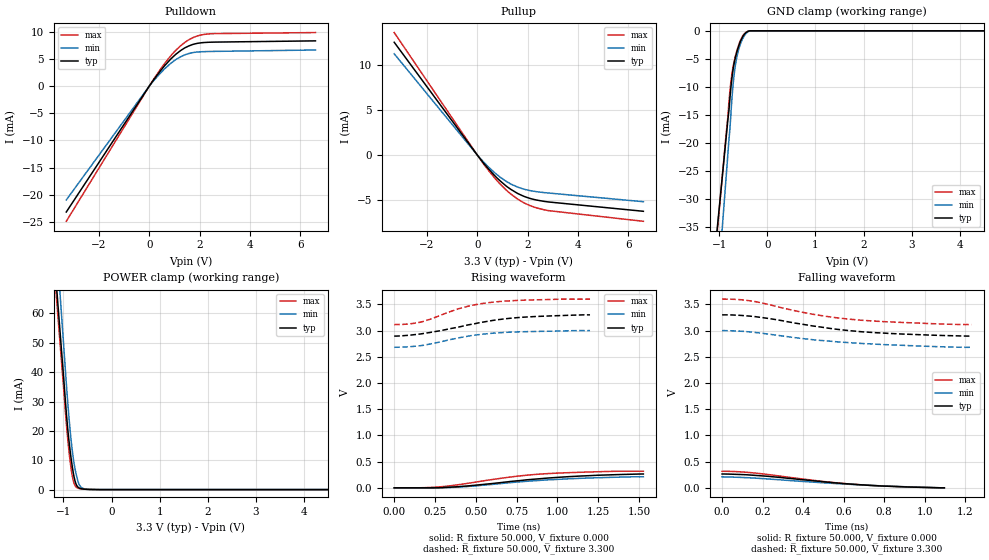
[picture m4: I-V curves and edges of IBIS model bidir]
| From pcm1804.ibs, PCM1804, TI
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[Model]   bidir
Model_type I/O
Vinl=8.000E-01
Vinh=2.000E+00
Vref=0.000E+00
Rref=1.000E+06
Cref=0.000E+00
Vmeas=1.650E+00
C_comp   8.900E-13   8.880E-13   8.930E-13
[Voltage Range]   3.300E+00   3.000E+00   3.600E+00
[POWER Clamp Reference]   3.300E+00   3.000E+00   3.600E+00
[GND Clamp Reference]   0.000E+00   0.000E+00   0.000E+00
[Pullup Reference]   3.300E+00   3.000E+00   3.600E+00
[Pulldown Reference]   0.000E+00   0.000E+00   0.000E+00
[Temperature Range]   25   70   -10
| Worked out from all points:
|   slope of the pulldown table from 0 to 0.495 V, typ, clamps not added: 160 ohm
|   slope of the pullup table from 0 to 0.495 V, typ, clamps not added: 292 ohm
|   GND clamp passes 1 mA (typ) near -0.51 V on its own axis
|   POWER clamp passes 1 mA (typ) near -0.71 V on its own axis
|   rising waveform, R_fixture 50.000, V_fixture 0.000: 20-80 % time 555ps typ, 530ps min, 454ps max; typ from 0 V to 0.264 V
|   falling waveform, R_fixture 50.000, V_fixture 0.000: 20-80 % time 459ps typ, 533ps min, 438ps max; typ from 0.264 V to 0 V
|   rising waveform, R_fixture 50.000, V_fixture 3.300: 20-80 % time 424ps typ, 337ps min, 298ps max; typ from 2.9 V to 3.3 V
|   falling waveform, R_fixture 50.000, V_fixture 3.300: 20-80 % time 445ps typ, 518ps min, 422ps max; typ from 3.3 V to 2.9 V
[GND Clamp]
-3.3V     -232.4mA   -302.2mA   -248.8mA
-860mV    -19.24mA   -26.33mA   -18.65mA
-820mV    -15.75mA   -21.82mA   -15.17mA
-800mV    -14.27mA   -19.5mA    -12.77mA
-780mV    -12.13mA   -17.61mA   -10.83mA
-760mV    -10.22mA   -15.02mA   -9.19mA
-720mV    -7.29mA    -10.23mA   -6.747mA
-660mV    -4.573mA   -5.874mA   -4.354mA
-560mV    -1.885mA   -2.334mA   -1.71mA
-480mV    -627.3uA   -874.5uA   -516.4uA
-400mV    -90.86uA   -152.2uA   -66.2uA
6.6V      0A         0A         0A
[Power Clamp]
-3.3V     522.9mA    587.4mA    513.2mA
-1.02V    43.15mA    54.89mA    39.38mA
-920mV    22.35mA    31.7mA     18.83mA
-880mV    15.84mA    23.62mA    12.3mA
-840mV    10.56mA    16.72mA    7.061mA
-800mV    6.176mA    11.23mA    3.341mA
-780mV    4.413mA    9.024mA    2.174mA
-740mV    1.98mA     5.539mA    938.8uA
-700mV    870.8uA    2.963mA    491.7uA
-620mV    272.2uA    601.8uA    212.3uA
-460mV    51.82uA    58.54uA    63.45uA
6.6V      0A         0A         0A
[Pullup]
-3.3V     12.56mA    11.28mA    13.64mA
20mV      -69.87uA   -65.87uA   -82.31uA
340mV     -1.204mA   -1.04mA    -1.32mA
700mV     -2.319mA   -1.99mA    -2.59mA
1.14V     -3.435mA   -2.915mA   -3.882mA
1.34V     -3.84mA    -3.241mA   -4.363mA
1.6V      -4.277mA   -3.569mA   -4.903mA
1.92V     -4.674mA   -3.856mA   -5.418mA
2.36V     -5.02mA    -4.089mA   -5.896mA
2.64V     -5.159mA   -4.183mA   -6.093mA
6.6V      -6.271mA   -5.204mA   -7.386mA
[Pulldown]
-3.3V     -23.19mA   -20.97mA   -24.9mA
120mV     803uA      694uA      882.4uA
480mV     3.018mA    2.567mA    3.335mA
800mV     4.717mA    3.968mA    5.266mA
1.06V     5.871mA    4.885mA    6.619mA
1.4V      6.994mA    5.719mA    7.996mA
1.7V      7.607mA    6.125mA    8.835mA
1.9V      7.85mA     6.255mA    9.209mA
2.36V     8.054mA    6.355mA    9.591mA
6.6V      8.311mA    6.63mA     9.839mA
[Rising Waveform]
R_fixture = 50.000
V_fixture = 0.000
V_fixture_min = 0.000
V_fixture_max = 0.000
|  time   V(typ)   V(min)   V(max)
0s        0V         0V         0V
177.5ps   0V         2.38uV     2.939mV
295ps     5.044mV    3.189mV    23.67mV
452.5ps   37.24mV    26.28mV    86.98mV
702.5ps   118.2mV    96.24mV    203mV
907.5ps   178.2mV    145.8mV    265.6mV
1.07ns    213.7mV    172.6mV    289.6mV
1.245ns   240mV      192.6mV    307.2mV
1.367ns   252.5mV    203.4mV    316.7mV
1.527ns   264.4mV    211.2mV    317.1mV
[Falling Waveform]
R_fixture = 50.000
V_fixture = 0.000
V_fixture_min = 0.000
V_fixture_max = 0.000
|  time   V(typ)   V(min)   V(max)
0s        264.4mV    211.2mV    317.1mV
82.5ps    255.9mV    200.7mV    307.1mV
152.5ps   241mV      188.1mV    286.3mV
232.5ps   218.1mV    167.9mV    251.3mV
457.5ps   132.4mV    107.1mV    140.6mV
550ps     97.82mV    84.85mV    101.4mV
647.5ps   68.31mV    64.06mV    68.22mV
760ps     41.25mV    42.63mV    41.76mV
852.5ps   25.49mV    28.29mV    27.12mV
1.097ns   0V         0V         0V
[Rising Waveform]
R_fixture = 50.000
V_fixture = 3.300
V_fixture_min = 3.000
V_fixture_max = 3.600
|  time   V(typ)   V(min)   V(max)
0s        2.895V     2.681V     3.115V
82.5ps    2.909V     2.69V      3.124V
162.5ps   2.936V     2.713V     3.162V
225ps     2.967V     2.747V     3.221V
395ps     3.067V     2.861V     3.417V
470ps     3.118V     2.903V     3.477V
567.5ps   3.174V     2.939V     3.529V
667.5ps   3.22V      2.963V     3.56V
790ps     3.255V     2.978V     3.58V
1.2ns     3.3V       3V         3.6V
[Falling Waveform]
R_fixture = 50.000
V_fixture = 3.300
V_fixture_min = 3.000
V_fixture_max = 3.600
|  time   V(typ)   V(min)   V(max)
0s        3.3V       3V         3.6V
80ps      3.292V     2.991V     3.592V
147.5ps   3.272V     2.97V      3.563V
267.5ps   3.208V     2.913V     3.461V
417.5ps   3.108V     2.839V     3.333V
517.5ps   3.05V      2.803V     3.269V
622.5ps   3.001V     2.771V     3.22V
865ps     2.938V     2.722V     3.159V
1.092ns   2.906V     2.69V      3.124V
1.23ns    2.895V     2.681V     3.115V
[Ramp]
dV/dt_r   1.5916E-01/5.5453E-10   1.2668E-01/5.3000E-10   1.9140E-01/4.5348E-10
dV/dt_f   2.4312E-01/4.4656E-10   1.9135E-01/5.1688E-10   2.9099E-01/4.1996E-10
R_load = 50
